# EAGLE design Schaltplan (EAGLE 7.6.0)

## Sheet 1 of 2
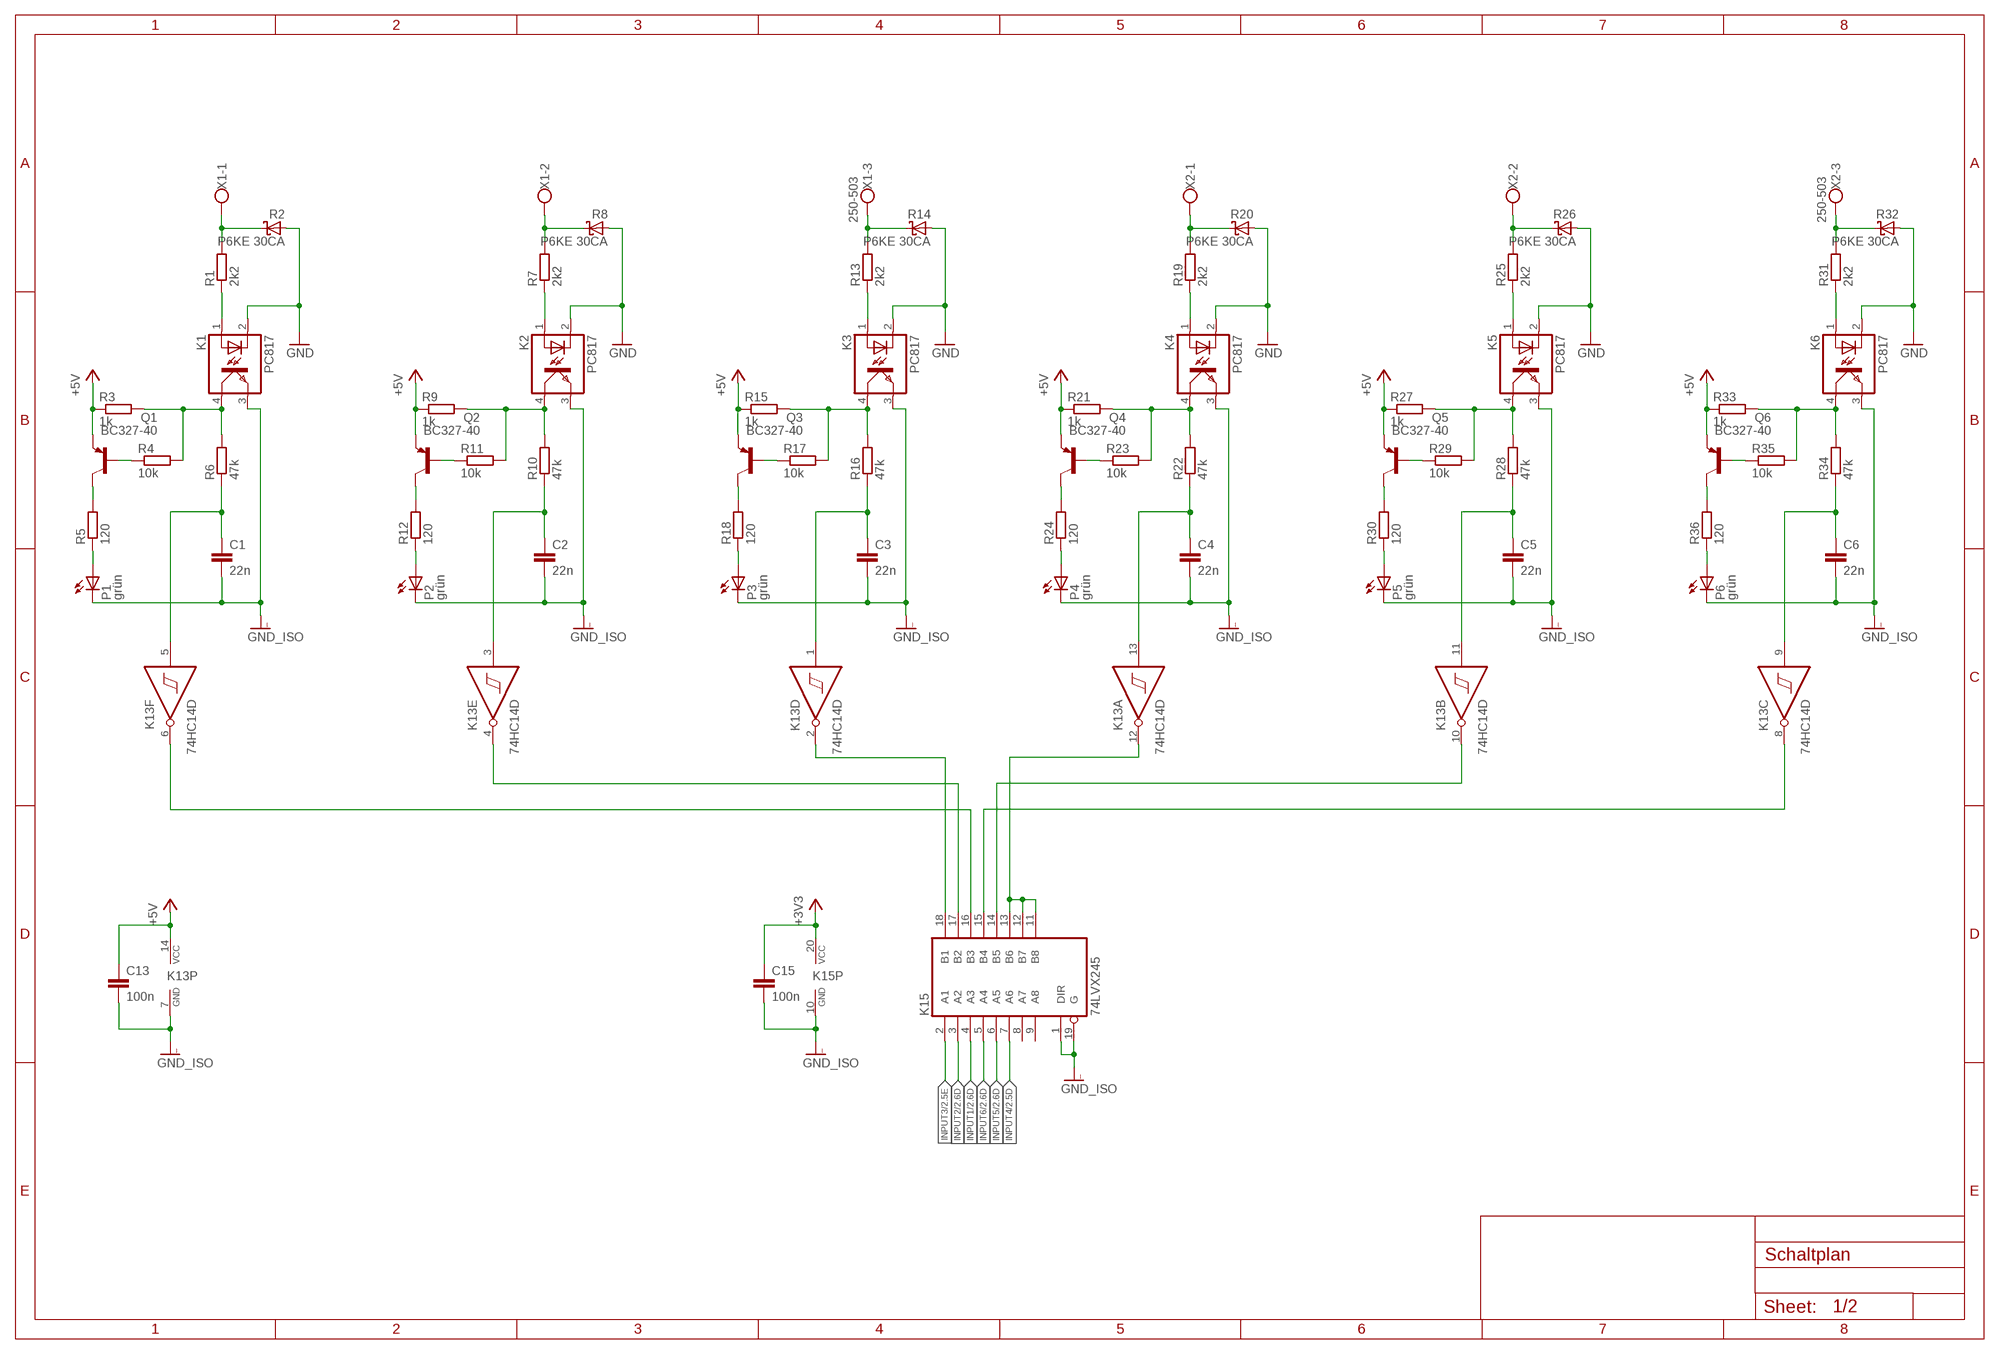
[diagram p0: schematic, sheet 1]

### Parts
C1  22n  C-EU025-024X044  [C025-024X044]
C2  22n  C-EU025-024X044  [C025-024X044]
C3  22n  C-EU025-024X044  [C025-024X044]
C4  22n  C-EU025-024X044  [C025-024X044]
C5  22n  C-EU025-024X044  [C025-024X044]
C6  22n  C-EU025-024X044  [C025-024X044]
C13  100n  C-EU025-024X044  [C025-024X044]
C15  100n  C-EU025-024X044  [C025-024X044]
K1  PC817  [DIL04]
K2  PC817  [DIL04]
K3  PC817  [DIL04]
K4  PC817  [DIL04]
K5  PC817  [DIL04]
K6  PC817  [DIL04]
K13  74HC14D  [SO14]
K15  74LVX245  74HCT245DW  [SO20W]
P1  grün  LED3MM  [LED3MM]
P2  grün  LED3MM  [LED3MM]
P3  grün  LED3MM  [LED3MM]
P4  grün  LED3MM  [LED3MM]
P5  grün  LED3MM  [LED3MM]
P6  grün  LED3MM  [LED3MM]
Q1  BC327-40  [TO92-EBC]
Q2  BC327-40  [TO92-EBC]
Q3  BC327-40  [TO92-EBC]
Q4  BC327-40  [TO92-EBC]
Q5  BC327-40  [TO92-EBC]
Q6  BC327-40  [TO92-EBC]
R1  2k2  R-EU_0207/12  [0207/12]
R2  P6KE 30CA  P6KEXX  [CB417-15]
R3  1k  R-EU_0207/7  [0207/7]
R4  10k  R-EU_0207/2V  [0207/2V]
R5  120  R-EU_0207/2V  [0207/2V]
R6  47k  R-EU_0207/2V  [0207/2V]
R7  2k2  R-EU_0207/12  [0207/12]
R8  P6KE 30CA  P6KEXX  [CB417-15]
R9  1k  R-EU_0207/7  [0207/7]
R10  47k  R-EU_0207/2V  [0207/2V]
R11  10k  R-EU_0207/2V  [0207/2V]
R12  120  R-EU_0207/2V  [0207/2V]
R13  2k2  R-EU_0207/12  [0207/12]
R14  P6KE 30CA  P6KEXX  [CB417-15]
R15  1k  R-EU_0207/7  [0207/7]
R16  47k  R-EU_0207/2V  [0207/2V]
R17  10k  R-EU_0207/2V  [0207/2V]
R18  120  R-EU_0207/2V  [0207/2V]
R19  2k2  R-EU_0207/12  [0207/12]
R20  P6KE 30CA  P6KEXX  [CB417-15]
R21  1k  R-EU_0207/7  [0207/7]
R22  47k  R-EU_0207/2V  [0207/2V]
R23  10k  R-EU_0207/2V  [0207/2V]
R24  120  R-EU_0207/2V  [0207/2V]
R25  2k2  R-EU_0207/12  [0207/12]
R26  P6KE 30CA  P6KEXX  [CB417-15]
R27  1k  R-EU_0207/7  [0207/7]
R28  47k  R-EU_0207/2V  [0207/2V]
R29  10k  R-EU_0207/2V  [0207/2V]
R30  120  R-EU_0207/2V  [0207/2V]
R31  2k2  R-EU_0207/12  [0207/12]
R32  P6KE 30CA  P6KEXX  [CB417-15]
R33  1k  R-EU_0207/7  [0207/7]
R34  47k  R-EU_0207/2V  [0207/2V]
R35  10k  R-EU_0207/2V  [0207/2V]
R36  120  R-EU_0207/2V  [0207/2V]
X1  250-503  W237-103  [W237-103]
X2  250-503  W237-103  [W237-103]

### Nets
+3V3: C15.1 K15.20(VCC) ; also sheet 2
+5V: C13.1 K13.14(P:VCC) Q1.E Q2.E Q3.E Q4.E Q5.E Q6.E R3.1 R9.1 R15.1 R21.1 R27.1 R33.1 ; also sheet 2
GND: K1.2(C) K2.2(C) K3.2(C) K4.2(C) K5.2(C) K6.2(C) R2.A R8.A R14.A R20.A R26.A R32.A ; also sheet 2
GNDI: C2.2 C3.2 C4.2 C5.2 C6.2 C13.2 C15.2 K2.3(EMIT) K3.3(EMIT) K4.3(EMIT) K5.3(EMIT) K6.3(EMIT) K13.7(P:GND) K15.1(DIR) K15.10(GND) K15.19(G) P2.K(C) P3.K(C) P4.K(C) P5.K(C) P6.K(C) ; supply symbol labelled GND_ISO ; also sheet 2
INPUT1: K15.4(A3) ; also sheet 2
INPUT2: K15.3(A2) ; also sheet 2
INPUT3: K15.2(A1) ; also sheet 2
INPUT4: K15.7(A6) ; also sheet 2
INPUT5: K15.6(A5) ; also sheet 2
INPUT6: K15.5(A4) ; also sheet 2
N$1: K1.1(A) R1.1
N$2: R7.2 R8.C X1.2
N$3: K2.1(A) R7.1
N$4: K2.4(COL) R9.2 R10.2 R11.2
N$8: R1.2 R2.C X1.1
N$9: Q2.B R11.1
N$10: Q2.C R12.2
N$11: P2.A R12.1
N$12: R13.2 R14.C X1.3
N$13: K3.1(A) R13.1
N$14: K3.4(COL) R15.2 R16.2 R17.2
N$15: Q3.B R17.1
N$16: Q1.C R5.2
N$17: K1.4(COL) R3.2 R4.2 R6.2
N$18: Q3.C R18.2
N$19: P1.A R5.1
N$23: Q1.B R4.1
N$24: P3.A R18.1
N$25: R19.2 R20.C X2.1
N$26: K4.1(A) R19.1
N$27: K4.4(COL) R21.2 R22.2 R23.2
N$28: Q4.B R23.1
N$29: Q4.C R24.2
N$30: P4.A R24.1
N$31: R25.2 R26.C X2.2
N$32: K5.1(A) R25.1
N$33: K5.4(COL) R27.2 R28.2 R29.2
N$34: Q5.B R29.1
N$35: Q5.C R30.2
N$36: P5.A R30.1
N$37: R31.2 R32.C X2.3
N$38: K6.1(A) R31.1
N$39: K6.4(COL) R33.2 R34.2 R35.2
N$40: Q6.B R35.1
N$41: Q6.C R36.2
N$42: P6.A R36.1
N$44: K13.2(D:O) K15.18(B1)
N$45: K13.4(E:O) K15.17(B2)
N$46: K13.6(F:O) K15.16(B3)
N$47: K13.12(A:O) K15.11(B8) K15.12(B7) K15.13(B6)
N$48: K13.10(B:O) K15.14(B5)
N$49: K13.8(C:O) K15.15(B4)
P!: C1.2 K1.3(EMIT) P1.K(C) ; supply symbol labelled GND_ISO
SIGNAL1: C1.1 K13.5(F:I) R6.1
SIGNAL2: C2.1 K13.3(E:I) R10.1
SIGNAL3: C3.1 K13.1(D:I) R16.1
SIGNAL4: C4.1 K13.13(A:I) R22.1
SIGNAL5: C5.1 K13.11(B:I) R28.1
SIGNAL6: C6.1 K13.9(C:I) R34.1
Unconnected: K15.8(A7) K15.9(A8)

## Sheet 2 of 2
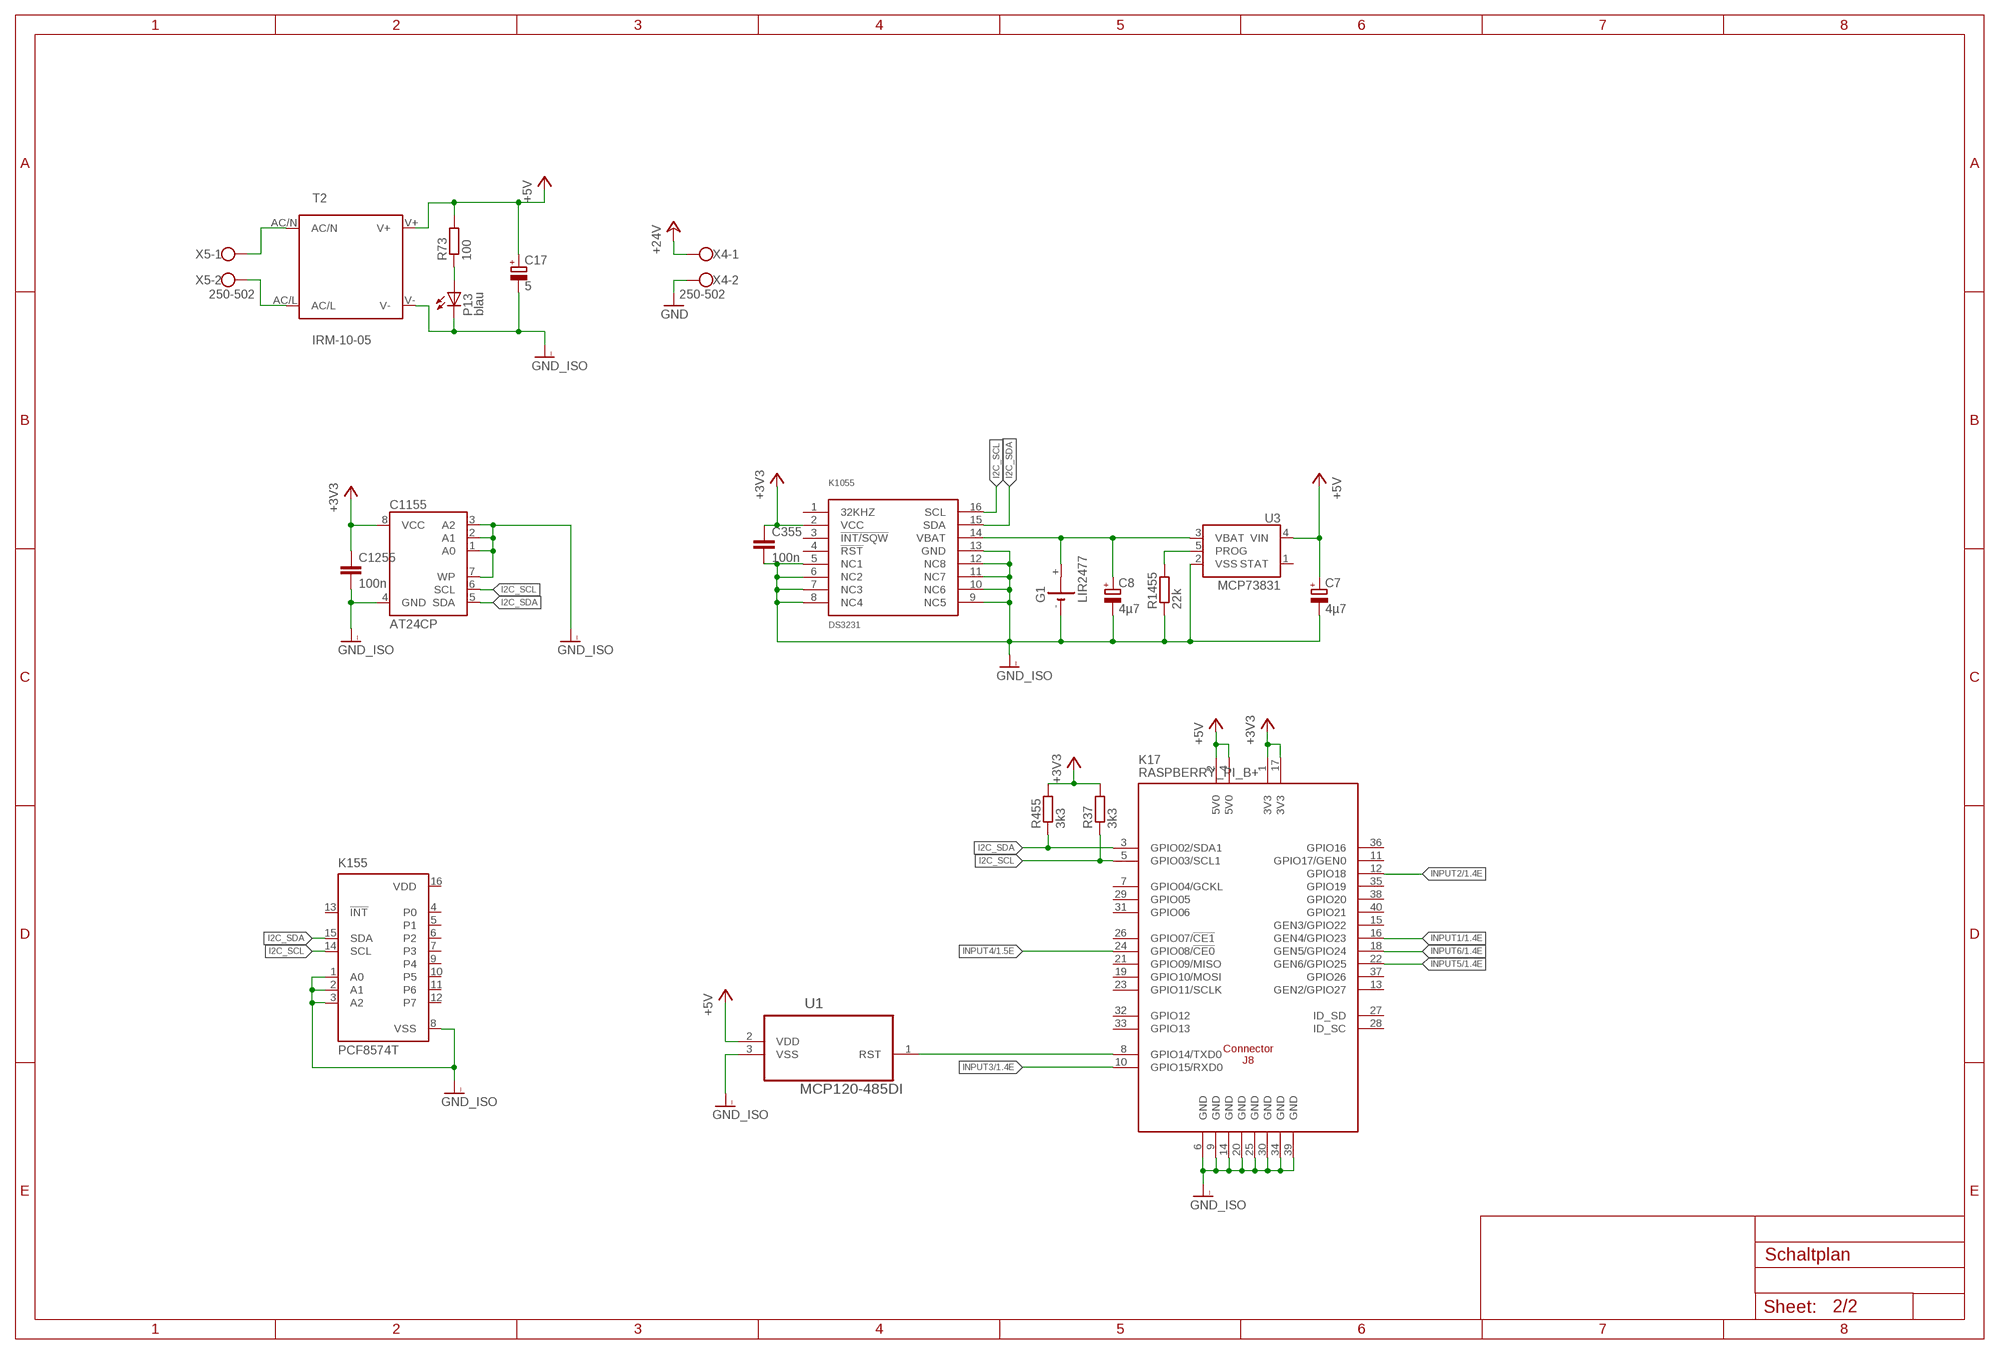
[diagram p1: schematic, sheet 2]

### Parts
C7  4µ7  CPOL-EUE2.5-5  [E2,5-5]
C8  4µ7  CPOL-EUE2.5-5  [E2,5-5]
C17  5  CPOL-EUE10-22.5  [EB22,5D]
C355  100n  C-EU025-025X050  [C025-025X050]
C1155  AT24CP  [DIL08]
C1255  100n  C-EU025-025X050  [C025-025X050]
G1  LIR2477  CR2430H  [CR2430H]
K17  RASPBERRY_PI_B+  [RASPBERRY_PI_BPLUS_NEU]
K155  PCF8574T  [SO16W]
K1055  DS3231  COMFILE_DS3231SN  [COMFILE_SO16W]
P13  blau  LED3MM  [LED3MM]
R37  3k3  R-EU_0207/5V  [0207/5V]
R73  100  R-EU_0207/7  [0207/7]
R455  3k3  R-EU_0207/2V  [0207/2V]
R1455  22k  R-EU_0207/7  [0207/7]
T2  IRM-10-05  IRM_05/10IRM_05/10  [IRM_05/10]
U1  MCP120-485DI  MCP120-300DI/TO  [TO127P254X495-3]
U3  MCP73831  [SOT23-5]
X4  250-502  W237-102  [W237-102]
X5  250-502  W237-102  [W237-102]

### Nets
+3V3: C355.1 C1155.8(VCC) C1255.1 K17.1(3V3) K17.17(3V3) K1055.2(VCC) R37.2 R455.2 ; also sheet 1
+5V: C7.+ C17.+ K17.2(5V0) K17.4(5V0) R73.2 T2.V+ U1.2(VDD) U3.4(VIN) ; also sheet 1
+24V: X4.1
GND: X4.2 ; also sheet 1
GND_ISO: K17.6(GND) K17.9(GND) K17.14(GND) K17.20(GND) K17.25(GND) K17.30(GND) K17.34(GND) K17.39(GND)
GNDI: C7.- C8.- C17.- C355.2 C1155.1(A0) C1155.2(A1) C1155.3(A2) C1155.4(GND) C1155.7(WP) C1255.2 G1.- K155.1(A0) K155.2(A1) K155.3(A2) K155.8(VSS) K1055.5(NC1) K1055.6(NC2) K1055.7(NC3) K1055.8(NC4) K1055.9(NC5) K1055.10(NC6) K1055.11(NC7) K1055.12(NC8) K1055.13(GND) P13.K(C) R1455.1 T2.V- U1.3(VSS) U3.2(VSS) ; supply symbol labelled GND_ISO ; also sheet 1
I2C_SCL: C1155.6(SCL) K17.5(GPIO03/SCL1) K155.14(SCL) K1055.16(SCL) R37.1
I2C_SDA: C1155.5(SDA) K17.3(GPIO02/SDA1) K155.15(SDA) K1055.15(SDA) R455.1
INPUT1: K17.16(GEN4/GPIO23) ; also sheet 1
INPUT2: K17.12(GPIO18) ; also sheet 1
INPUT3: K17.10(GPIO15/RXD0) ; also sheet 1
INPUT4: K17.24(GPIO08/!CE0!) ; also sheet 1
INPUT5: K17.22(GEN6/GPIO25) ; also sheet 1
INPUT6: K17.18(GEN5/GPIO24) ; also sheet 1
N$20: R1455.2 U3.5(PROG)
N$50: K17.8(GPIO14/TXD0) U1.1(RST)
N$91: P13.A R73.1
N$92: T2.AC/N X5.1
N$93: T2.AC/L X5.2
VBAT: C8.+ G1.+ K1055.14(VBAT) U3.3(VBAT)
Unconnected: G1.+@1(+) K17.7(GPIO04/GCKL) K17.11(GPIO17/GEN0) K17.13(GEN2/GPIO27) K17.15(GEN3/GPIO22) K17.19(GPIO10/MOSI) K17.21(GPIO09/MISO) K17.23(GPIO11/SCLK) K17.26(GPIO07/!CE1!) K17.27(ID_SD) K17.28(ID_SC) K17.29(GPIO05) K17.31(GPIO06) K17.32(GPIO12) K17.33(GPIO13) K17.35(GPIO19) K17.36(GPIO16) K17.37(GPIO26) K17.38(GPIO20) K17.40(GPIO21) K155.4(P0) K155.5(P1) K155.6(P2) K155.7(P3) K155.9(P4) K155.10(P5) K155.11(P6) K155.12(P7) K155.13(!INT) K1055.1(32KHZ) K1055.3(!INT/SQW) K1055.4(!RST) U3.1(STAT)

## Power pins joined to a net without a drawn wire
VDD: K155.16(VDD)

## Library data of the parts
C1-C6 C13 C15 C355 C1255 = resistor:C-EU: CAPACITOR, European symbol
C7 C8 C17 = resistor:CPOL-EU: POLARIZED CAPACITOR, European symbol
C1155 = atmel:AT24C*: 2-wire serial EEPROM; MPN: AT24C1024BW-SH-B; OC_FARNELL: 1362646; OC_NEWARK: 03P2044
G1 = battery:CR2430H: LI BATTERY Varta
K1-K6 = optocoupler:PC817: SHARP OPTO COUPLER; MPN: PC817X4J000F; OC_FARNELL: 9707727; OC_NEWARK: 97K7059
K13 = 74xx-eu:74*14: Hex schmitt trigger INVERTER
K15 = 74xx-eu:74*245: Octal BUS TRANSCEIVER, 3-state
K17 = RASPBERRY_PI_Bplus:RASPBERRY_PI_B+: Raspberry Pi B+ Basedon issue: Thursday, July 10, 2014 - Rev 1.2 LBR by Tim Rettmann 07-2014
K155 = micro-philips:PCF8574: I2C-Bus Remote 8-bit I/O expander http://www.semiconductors.philips.com/acrobat_download/datasheets/PCF8574_4.pdf; MPN: PCF8574T/3,512; OC_FARNELL: 1201255; OC_NEWARK: 70R6870
K1055 = board:COMFILE_DS3231SN
P1-P6 P13 = led:LED: LED
Q1-Q6 = transistor-pnp:BC327*: PNP Transistror
R1 R3-R7 R9-R13 R15-R19 R21-R25 R27-R31 R33-R37 R73 R455 R1455 = resistor:R-EU_: RESISTOR, European symbol
R2 R8 R14 R20 R26 R32 = diode:P6KEXX: DIODE
T2 = meanwell_irm_v7:IRM_05/10: 5 or 10 watt housing & pin compatible IRM 05 Vout [V] Imax [A] Pmax [W] Eff [%] 3.3 1.25 4.125 68 5 1 5 71 12 0.42 5.04 75 15 0.33 4.95 75 24 0.23 5.52 77 IRM 10 Vout [V] Imax [A] Pmax [W] Eff [%] 3.3 2.5 8.25 74 5 2 10 77 12 0.85 10.2 82 15 0.67 10.05 82 24 0.42 10.08 82
U1 = Microchip_By_element14_Batch_1:MCP120-300DI/TO: SUPERVISOR, OPEN DRAIN, SMD, TO-92; MPN: MCP120-300DI/TO; OC_FARNELL: 1332063; OC_NEWARK: 19C7145; PACKAGE: TO-92; SUPPLIER: Microchip
U3 = SparkFun:MCP73831: Microchip's MCP73831 Miniature single cell, fully integrated Li-Ion, Li-polymer charge management controller http://ww1.microchip.com/downloads/en/DeviceDoc/21984a.pdf
X1 X2 = con-wago-500:W237-103: WAGO SCREW CLAMP; MPN: 237-103; OC_FARNELL: unknown; OC_NEWARK: 18M7116
X4 X5 = con-wago-500:W237-102: WAGO SCREW CLAMP; MPN: 237-102; OC_FARNELL: unknown; OC_NEWARK: 70K9898

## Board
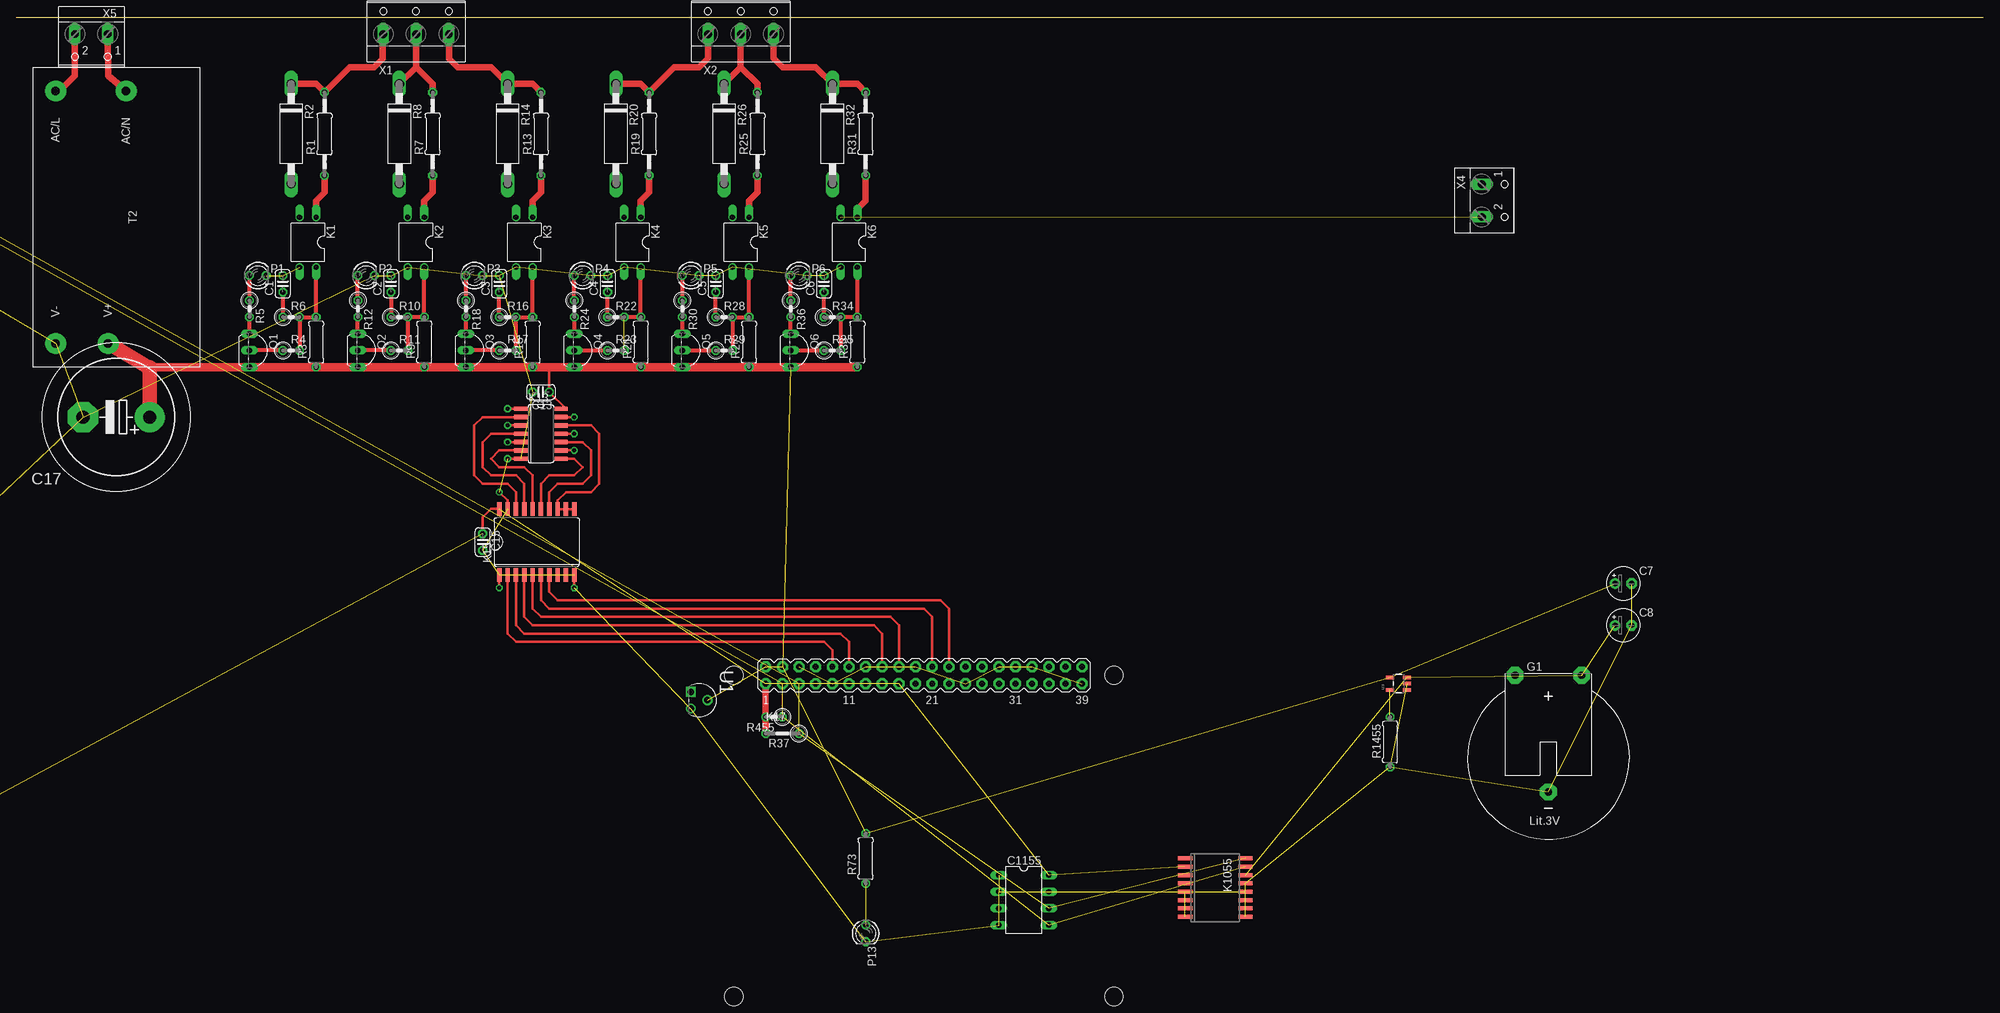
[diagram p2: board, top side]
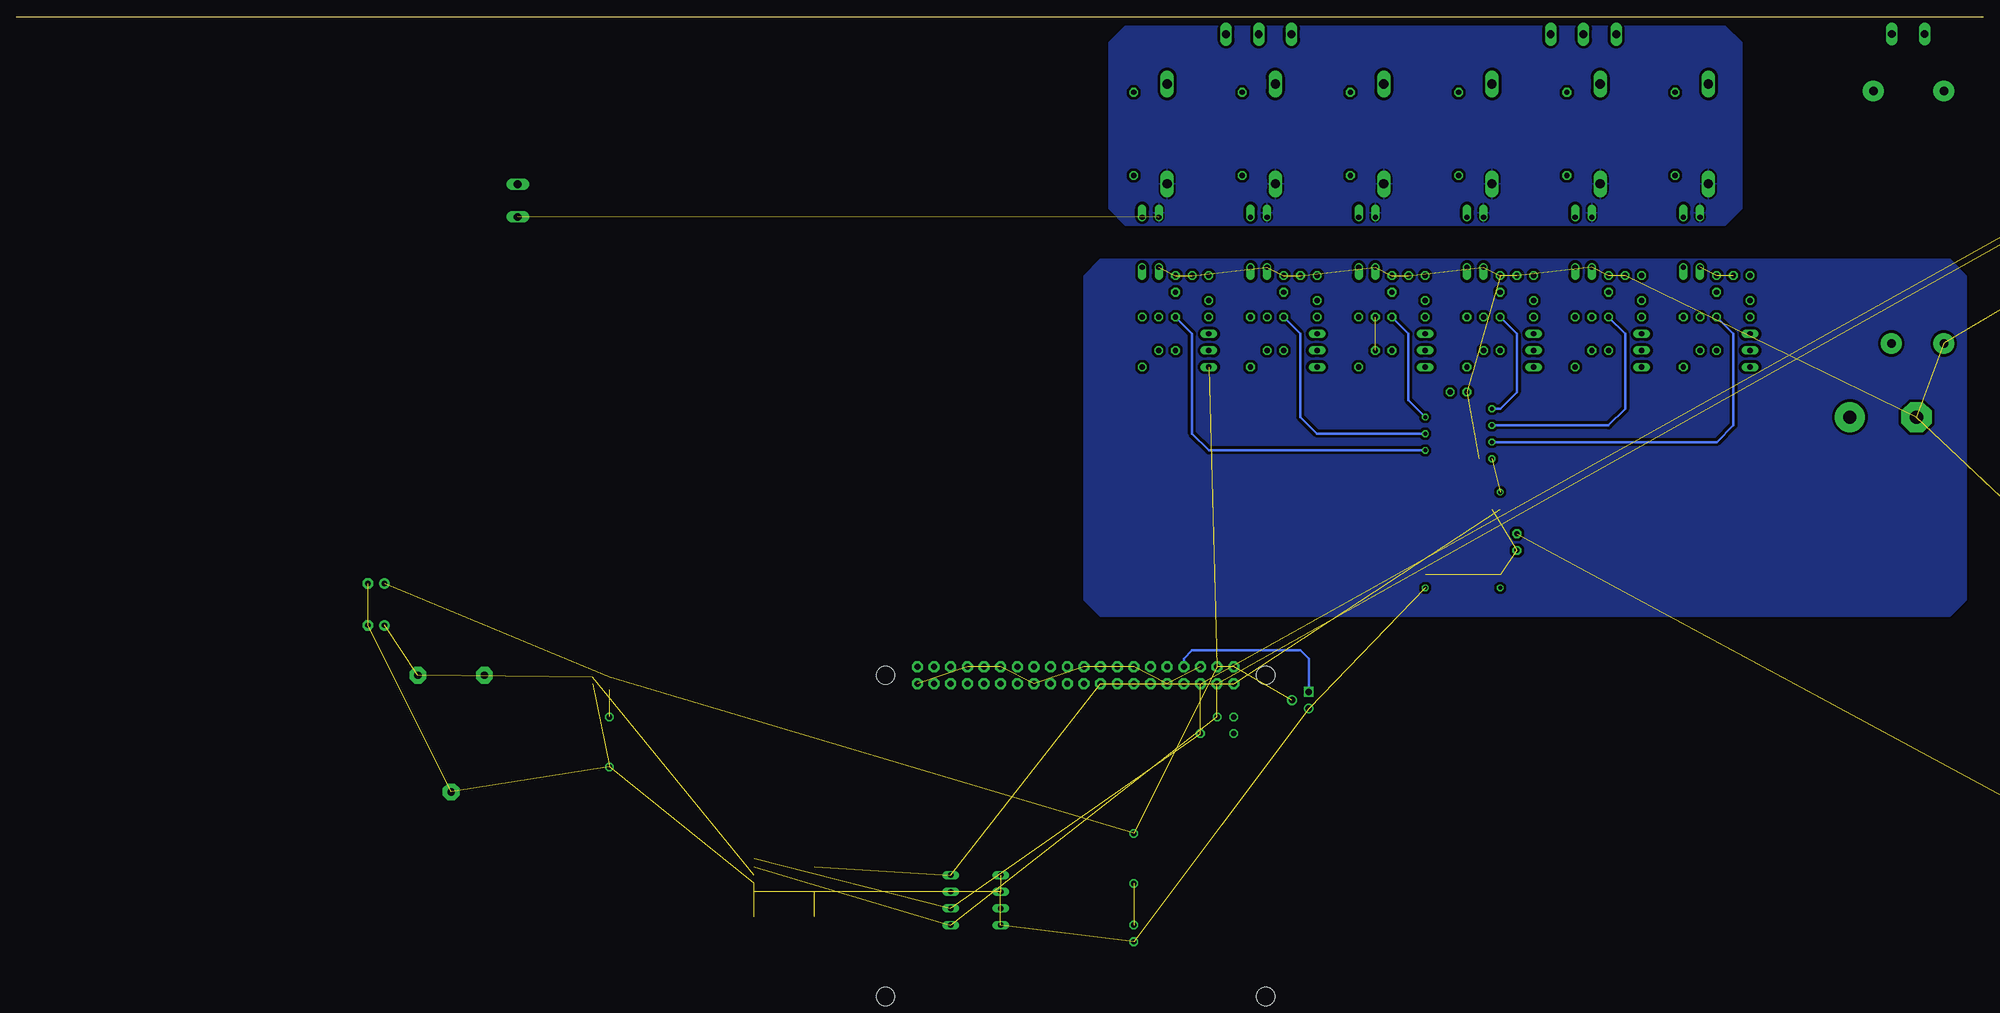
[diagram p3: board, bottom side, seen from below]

Size 300 x 0 mm. Coordinates in mm from the lower left corner, seen from the top.
Outline: 0,0 300,0
Copper layers (1*16): Top 0.035mm / dielectric 2mm / Bottom 0.035mm
Design rules "default *": minimum track width 10mil, minimum drill 24mil, track to track 8mil, track to pad 8mil, pad to pad 8mil, via to via 8mil, smd to smd 8mil, copper to edge 40mil, drill to drill 8mil, minimum pad ring 10mil, minimum via ring 8mil, stop-mask expansion 4mil, vias tented up to drill 0mil, thermal gap 10mil

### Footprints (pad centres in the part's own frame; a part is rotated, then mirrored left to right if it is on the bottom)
C025-024X044 = drill 0.813 octagon: 1 -1.27,0; 2 1.27,0
E2,5-5 = drill 0.813 pad 1.6: + -1.27,0 | drill 0.813 pad 1.6 octagon: - 1.27,0
EB22,5D = drill 2.007 pad 4.597: + -5.08,0 | drill 2.007 pad 4.597 octagon: - 5.08,0
C025-025X050 = drill 0.813 octagon: 1 -1.27,0; 2 1.27,0
DIL08 = drill 0.813 long: 1 -3.81,-3.81; 2 -1.27,-3.81; 3 1.27,-3.81; 4 3.81,-3.81; 5 3.81,3.81; 6 1.27,3.81; 7 -1.27,3.81; 8 -3.81,3.81
CR2430H = drill 1.118 pad 2.54 octagon: + 5.08,12.7; +@1 -5.08,12.7; - 0,-5.08
DIL04 = drill 0.813 offset: 1 -1.27,-3.81; 2 1.27,-3.81; 3 1.27,3.81; 4 -1.27,3.81
SO14 = smd 0.66 x 2.032: 1 -3.81,-3.073; 2 -2.54,-3.073; 3 -1.27,-3.073; 4 0,-3.073; 5 1.27,-3.073; 6 2.54,-3.073; 7 3.81,-3.073; 8 3.81,3.073; 9 2.54,3.073; 10 1.27,3.073; 11 0,3.073; 12 -1.27,3.073; 13 -2.54,3.073; 14 -3.81,3.073
SO20W = smd 0.66 x 2.032: 1 -5.715,-5.029; 2 -4.445,-5.029; 3 -3.175,-5.029; 4 -1.905,-5.029; 5 -0.635,-5.029; 6 0.635,-5.029; 7 1.905,-5.029; 8 3.175,-5.029; 9 4.445,-5.029; 10 5.715,-5.029; 11 5.715,5.029; 12 4.445,5.029; 13 3.175,5.029; 14 1.905,5.029; 15 0.635,5.029; 16 -0.635,5.029; 17 -1.905,5.029; 18 -3.175,5.029; 19 -4.445,5.029; 20 -5.715,5.029
RASPBERRY_PI_BPLUS_NEU = drill 0.9 pad 1.676 octagon: 1 -24.13,-1.27; 2 -24.13,1.27; 3 -21.59,-1.27; 4 -21.59,1.27; 5 -19.05,-1.27; 6 -19.05,1.27; 7 -16.51,-1.27; 8 -16.51,1.27; 9 -13.97,-1.27; 10 -13.97,1.27; 11 -11.43,-1.27; 12 -11.43,1.27; 13 -8.89,-1.27; 14 -8.89,1.27; 15 -6.35,-1.27; 16 -6.35,1.27; 17 -3.81,-1.27; 18 -3.81,1.27; 19 -1.27,-1.27; 20 -1.27,1.27; 21 1.27,-1.27; 22 1.27,1.27; 23 3.81,-1.27; 24 3.81,1.27; 25 6.35,-1.27; 26 6.35,1.27; 27 8.89,-1.27; 28 8.89,1.27; 29 11.43,-1.27; 30 11.43,1.27; 31 13.97,-1.27; 32 13.97,1.27; 33 16.51,-1.27; 34 16.51,1.27; 35 19.05,-1.27; 36 19.05,1.27; 37 21.59,-1.27; 38 21.59,1.27; 39 24.13,-1.27; 40 24.13,1.27 | hole 2.8: -29,0; 29,0; -29,-49; 29,-49
SO16W = smd 0.6 x 2.2: 1 -4.445,-4.6; 2 -3.175,-4.6; 3 -1.905,-4.6; 4 -0.635,-4.6; 5 0.635,-4.6; 6 1.905,-4.6; 7 3.175,-4.6; 8 4.445,-4.6; 9 4.445,4.6; 10 3.175,4.6; 11 1.905,4.6; 12 0.635,4.6; 13 -0.635,4.6; 14 -1.905,4.6; 15 -3.175,4.6; 16 -4.445,4.6
COMFILE_SO16W = smd 0.6 x 2.2: 1 -4.445,-4.6; 2 -3.175,-4.6; 3 -1.905,-4.6; 4 -0.635,-4.6; 5 0.635,-4.6; 6 1.905,-4.6; 7 3.175,-4.6; 8 4.445,-4.6; 9 4.445,4.6; 10 3.175,4.6; 11 1.905,4.6; 12 0.635,4.6; 13 -0.635,4.6; 14 -1.905,4.6; 15 -3.175,4.6; 16 -4.445,4.6
LED3MM = drill 0.813 octagon: A -1.27,0; K 1.27,0
TO92-EBC = drill 0.813 long: B 0,-1.27; C -2.54,-1.27; E 2.54,-1.27
0207/12 = drill 0.813 octagon: 1 -6.35,0; 2 6.35,0
CB417-15 = drill 1.397 long: A 7.62,0; C -7.62,0
0207/7 = drill 0.813 octagon: 1 -3.81,0; 2 3.81,0
0207/2V = drill 0.813 octagon: 1 -1.27,0; 2 1.27,0
0207/5V = drill 0.813 octagon: 1 -2.54,0; 2 2.54,0
IRM_05/10 = drill 1.3 pad 3.17: AC/L -19.25,-9.25; AC/N -19.25,1.5; V+ 19.25,-1.25; V- 19.25,-9.25
TO127P254X495-3 = drill 0.991 square: 1 -2.54,-2.54 | drill 0.991: 2 -1.27,0; 3 0,-2.54
SOT23-5 = smd 0.55 x 1.2: 1 -0.95,-1.3; 2 0,-1.3; 3 0.95,-1.3; 4 0.95,1.3; 5 -0.95,1.3
W237-103 = drill 1.194 long: 1 -5,-1.29; 2 0,-1.29; 3 5,-1.29
W237-102 = drill 1.194 long: 1 -2.5,-1.27; 2 2.5,-1.27

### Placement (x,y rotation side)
C1  40.64,-40.64 90 top  (outside the outline)
C2  57.15,-40.64 90 top  (outside the outline)
C3  73.66,-40.64 90 top  (outside the outline)
C4  90.17,-40.64 90 top  (outside the outline)
C5  106.68,-40.64 90 top  (outside the outline)
C6  123.19,-40.64 90 top  (outside the outline)
C7  not placed on the board
C8  not placed on the board
C13  80.01,-57.15 180 top  (outside the outline)
C15  71.12,-80.01 270 top  (outside the outline)
C17  15.24,-60.96 180 top  (outside the outline)
C355  not placed on the board
C1155  not placed on the board
C1255  not placed on the board
G1  not placed on the board
K1  44.45,-34.29 180 top  (outside the outline)
K2  60.96,-34.29 180 top  (outside the outline)
K3  77.47,-34.29 180 top  (outside the outline)
K4  93.98,-34.29 180 top  (outside the outline)
K5  110.49,-34.29 180 top  (outside the outline)
K6  127,-34.29 180 top  (outside the outline)
K13  80.01,-63.5 270 top  (outside the outline)
K15  79.38,-80.01 0 top  (outside the outline)
K17  138.43,-100.33 0 top  (outside the outline)
K155  not placed on the board
K1055  not placed on the board
P1  36.83,-39.37 0 top  (outside the outline)
P2  53.34,-39.37 0 top  (outside the outline)
P3  69.85,-39.37 0 top  (outside the outline)
P4  86.36,-39.37 0 top  (outside the outline)
P5  102.87,-39.37 0 top  (outside the outline)
P6  119.38,-39.37 0 top  (outside the outline)
P13  not placed on the board
Q1  36.83,-50.8 270 top  (outside the outline)
Q2  53.34,-50.8 270 top  (outside the outline)
Q3  69.85,-50.8 270 top  (outside the outline)
Q4  86.36,-50.8 270 top  (outside the outline)
Q5  102.87,-50.8 270 top  (outside the outline)
Q6  119.38,-50.8 270 top  (outside the outline)
R1  46.99,-17.78 90 top  (outside the outline)
R2  41.91,-17.78 270 top  (outside the outline)
R3  45.72,-49.53 90 top  (outside the outline)
R4  41.91,-50.8 0 top  (outside the outline)
R5  35.56,-44.45 270 top  (outside the outline)
R6  41.91,-45.72 0 top  (outside the outline)
R7  63.5,-17.78 90 top  (outside the outline)
R8  58.42,-17.78 270 top  (outside the outline)
R9  62.23,-49.53 90 top  (outside the outline)
R10  58.42,-45.72 0 top  (outside the outline)
R11  58.42,-50.8 0 top  (outside the outline)
R12  52.07,-44.45 270 top  (outside the outline)
R13  80.01,-17.78 90 top  (outside the outline)
R14  74.93,-17.78 270 top  (outside the outline)
R15  78.74,-49.53 90 top  (outside the outline)
R16  74.93,-45.72 0 top  (outside the outline)
R17  74.93,-50.8 0 top  (outside the outline)
R18  68.58,-44.45 270 top  (outside the outline)
R19  96.52,-17.78 90 top  (outside the outline)
R20  91.44,-17.78 270 top  (outside the outline)
R21  95.25,-49.53 90 top  (outside the outline)
R22  91.44,-45.72 0 top  (outside the outline)
R23  91.44,-50.8 0 top  (outside the outline)
R24  85.09,-44.45 270 top  (outside the outline)
R25  113.03,-17.78 90 top  (outside the outline)
R26  107.95,-17.78 270 top  (outside the outline)
R27  111.76,-49.53 90 top  (outside the outline)
R28  107.95,-45.72 0 top  (outside the outline)
R29  107.95,-50.8 0 top  (outside the outline)
R30  101.6,-44.45 270 top  (outside the outline)
R31  129.54,-17.78 90 top  (outside the outline)
R32  124.46,-17.78 270 top  (outside the outline)
R33  128.27,-49.53 90 top  (outside the outline)
R34  124.46,-45.72 0 top  (outside the outline)
R35  124.46,-50.8 0 top  (outside the outline)
R36  118.11,-44.45 270 top  (outside the outline)
R37  116.84,-109.22 180 top  (outside the outline)
R73  not placed on the board
R455  115.57,-106.68 180 top  (outside the outline)
R1455  not placed on the board
T2  15.24,-30.48 270 top  (outside the outline)
U1  105.41,-105.41 270 top  (outside the outline)
U3  not placed on the board
X1  60.96,-1.27 0 top
X2  110.49,-1.27 0 top
X4  not placed on the board
X5  11.43,-3.81 180 top

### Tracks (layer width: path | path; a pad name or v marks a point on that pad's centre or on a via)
+3V3  (6 unrouted)
  Top 0.406: C15.1 71.12,-76.2 72.39,-74.93 73.61,-74.93 K15.20
  Top 1.016: K17.1 R455.2 R37.2
+5V  (6 unrouted)
  Top 0.406: 81.28,-53.34 C13.1 83.82,-59.69 K13.14
  Top 1.016: 20.32,-53.34 20.14,-53.34
  Top 1.27: 20.32,-53.34 Q1.E R3.1 Q2.E R9.1 Q3.E R15.1 81.28,-53.34 Q4.E R21.1 Q5.E R27.1 Q6.E R33.1
  Top 2.184: 20.14,-53.34 T2.V+ | C17.+ 20.32,-53.34
GND  (1 unrouted)
  pour Bottom (isolate 0.406): 36.83,-29.21 39.37,-31.75 130.81,-31.75 133.35,-29.21 133.35,-3.81 130.81,-1.27 39.37,-1.27 36.83,-3.81
GND_ISO  (7 unrouted)
  pour Bottom (isolate 0.406): 43.18,-36.83 5.08,-36.83 2.54,-39.37 2.54,-88.9 5.08,-91.44 134.62,-91.44 137.16,-88.9 137.16,-39.37 134.62,-36.83
GNDI  (49 unrouted)
  Top 0.406: K13.7 74.93,-67.31 | K15.19 74.93,-73.66 73.66,-72.39 | K15.1 73.66,-87 | K15.10 85.09,-87
I2C_SCL  (4 unrouted)
I2C_SDA  (4 unrouted)
INPUT1
  Top 0.406: K15.4 77.47,-91.44 78.74,-92.71 130.81,-92.71 132.08,-93.98 K17.16
INPUT2
  Top 0.406: K15.3 76.2,-92.71 77.47,-93.98 125.73,-93.98 127,-95.25 K17.12
INPUT3
  Top 0.406: K15.2 74.93,-93.98 76.2,-95.25 123.19,-95.25 124.46,-96.52 K17.10
INPUT4
  Top 0.406: K15.7 81.28,-87.63 82.55,-88.9 140.97,-88.9 142.24,-90.17 K17.24
INPUT5
  Top 0.406: K15.6 80.01,-88.9 81.28,-90.17 138.43,-90.17 139.7,-91.44 K17.22
INPUT6
  Top 0.406: K15.5 78.74,-90.17 80.01,-91.44 133.35,-91.44 134.62,-92.71 K17.18
N$1
  Top 1.016: R1.1 46.99,-26.67 45.72,-27.94 K1.1
N$2
  Top 1.016: X1.2 60.96,-7.62 | 60.96,-7.62 R8.C | R7.2 63.5,-10.16 60.96,-7.62
N$3
  Top 1.016: R7.1 63.5,-26.67 62.23,-27.94 K2.1
N$4
  Top 0.61: K2.4 R9.2 R10.2 R11.2
N$5  (via drill 0.6)
  other vias: 74.93,-67.31
N$6  (via drill 0.6)
  other vias: 73.66,-87
N$7  (via drill 0.6)
  other vias: 85.09,-87
N$8
  Top 1.016: R2.C 45.72,-10.16 R1.2 50.8,-7.62 54.61,-7.62 55.88,-6.35 55.88,-2.64 X1.1
N$9
  Top 0.61: R11.1 Q2.B
N$10
  Top 0.61: Q2.C R12.2
N$11
  Top 0.61: R12.1 P2.A
N$12
  Top 1.016: R13.2 78.74,-10.16 R14.C 72.39,-7.62 67.31,-7.62 66.04,-6.35 66.04,-2.54 65.98,-2.54 X1.3
N$13
  Top 1.016: R13.1 80.01,-26.67 78.74,-27.94 K3.1
N$14
  Top 0.61: R17.2 R16.2 R15.2 K3.4
N$15
  Top 0.61: R17.1 Q3.B
N$16
  Top 0.61: Q1.C R5.2
N$17
  Top 0.61: K1.4 R3.2 R6.2 R4.2
N$18
  Top 0.61: Q3.C R18.2
N$19
  Top 0.61: R5.1 P1.A
N$20  (1 unrouted)
N$23
  Top 0.61: R4.1 Q1.B
N$24
  Top 0.61: R18.1 P3.A
N$25
  Top 1.016: R20.C 95.25,-10.16 R19.2 100.33,-7.62 104.14,-7.62 105.49,-6.27 X2.1
N$26
  Top 1.016: R19.1 96.52,-26.67 95.25,-27.94 K4.1
N$27  (1 unrouted)
  Top 0.61: R22.2 R21.2 K4.4
N$28
  Top 0.61: Q4.B R23.1
N$29
  Top 0.61: R24.2 Q4.C
N$30
  Top 0.61: R24.1 P4.A
N$31
  Top 1.016: R26.C 110.49,-7.62 | 110.49,-7.62 X2.2 | R25.2 113.03,-10.16 110.49,-7.62
N$32
  Top 1.016: R25.1 113.03,-26.67 111.76,-27.94 K5.1
N$33
  Top 0.61: K5.4 R27.2 R28.2 R29.2
N$34
  Top 0.61: Q5.B R29.1
N$35
  Top 0.61: Q5.C R30.2
N$36
  Top 0.61: R30.1 P5.A
N$37
  Top 1.016: X2.3 115.49,-6.27 116.84,-7.62 121.92,-7.62 R32.C 128.27,-10.16 R31.2
N$38
  Top 1.016: R31.1 129.54,-27.94 128.27,-29.21 K6.1
N$39
  Top 0.61: R35.2 R34.2 R33.2 K6.4
N$40
  Top 0.61: Q6.B R35.1
N$41
  Top 0.61: Q6.C R36.2
N$42
  Top 0.61: R36.1 P6.A
N$43  (via drill 0.6)
  other vias: 73.66,-72.39
N$44
  Top 0.406: K13.2 71.12,-60.96 69.85,-62.23 69.85,-69.85 71.12,-71.12 74.93,-71.12 76.2,-72.39 K15.18
N$45
  Top 0.406: K13.4 72.39,-63.5 71.12,-64.77 71.12,-68.58 72.39,-69.85 76.2,-69.85 77.47,-71.12 K15.17
N$46
  Top 0.406: K13.6 73.66,-66.04 72.39,-67.31 73.66,-68.58 77.47,-68.58 78.74,-69.85 K15.16
N$47
  Top 0.406: K13.12 87.63,-62.23 88.9,-63.5 88.9,-71.12 87.63,-72.39 83.82,-72.39 82.55,-73.66 K15.13 K15.12 K15.11
N$48
  Top 0.406: K13.10 86.36,-64.77 87.63,-66.04 87.63,-69.85 86.36,-71.12 82.55,-71.12 81.28,-72.39 K15.14
N$49
  Top 0.406: K13.8 85.09,-67.31 86.36,-68.58 85.09,-69.85 81.28,-69.85 80.01,-71.12 K15.15
N$50
  Bottom 0.406: U1.1 102.87,-97.79 104.14,-96.52 120.65,-96.52 121.92,-97.79 K17.8
N$91  (1 unrouted)
N$92
  Top 1.016: X5.1 13.97,-8.89 T2.AC/N
N$93
  Top 1.016: X5.2 8.89,-2.54 8.89,-8.89 6.35,-11.43 6.19,-11.43 T2.AC/L
P!  (2 unrouted)
SIGNAL1  (via drill 0.6)
  Top 0.406: v74.93,-64.77 K13.5
  Top 0.61: C1.1 R6.1
  Bottom 0.406: R6.1 38.1,-48.26 38.1,-62.23 40.64,-64.77 v74.93,-64.77
SIGNAL2  (via drill 0.6)
  Top 0.406: v74.93,-62.23 K13.3
  Top 0.61: C2.1 R10.1
  Bottom 0.406: R10.1 54.61,-48.26 54.61,-59.69 57.15,-62.23 v74.93,-62.23
SIGNAL3  (via drill 0.6)
  Top 0.406: v74.93,-59.69 K13.1
  Top 0.61: R16.1 C3.1
  Bottom 0.406: R16.1 71.12,-48.26 71.12,-57.15 73.66,-59.69 v74.93,-59.69
SIGNAL4  (via drill 0.6)
  Top 0.406: K13.13 v85.09,-60.96
  Top 0.61: R22.1 C4.1
  Bottom 0.406: R22.1 87.63,-48.26 87.63,-58.42 v85.09,-60.96
SIGNAL5  (via drill 0.6)
  Top 0.406: K13.11 v85.09,-63.5
  Top 0.61: R28.1 C5.1
  Bottom 0.406: R28.1 104.14,-48.26 104.14,-60.96 101.6,-63.5 v85.09,-63.5
SIGNAL6  (via drill 0.6)
  Top 0.406: K13.9 v85.09,-66.04
  Top 0.61: R34.1 C6.1
  Bottom 0.406: R34.1 120.65,-48.26 120.65,-63.5 118.11,-66.04 v85.09,-66.04
VBAT  (3 unrouted)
